(* Logix 5000 AddOnInstructionDefinition export AMCI_5034_PTO_AM_Preset_Encoder; software revision 37.00 *)

TYPE AMCI_5034_PTO_AM_Input_Data :
STRUCT
   ConnectionFaulted : DINT;
   MovingCW : BOOL;
   MovingCCW : BOOL;
   InHoldState : BOOL;
   Stopped : BOOL;
   AtHome : BOOL;
   Accelerating : BOOL;
   Decelerating : BOOL;
   MoveComplete : BOOL;
   HomeInvalid : BOOL;
   InvalidProfile : BOOL;
   PositionInvalid : BOOL;
   InputError : BOOL;
   CommandError : BOOL;
   ConfigurationError : BOOL;
   ModuleOK : BOOL;
   GeneralPurposeOutputStatus : BOOL;
   Input1Active : BOOL;
   Input2Active : BOOL;
   Input3Active : BOOL;
   Input4Active : BOOL;
   bit_20_reserved : BOOL;
   bit_21_reserved : BOOL;
   bit_22_reserved : BOOL;
   EncoderFollowerMode : BOOL;
   BlendMoveRunning : BOOL;
   BlendMoveAcknowledge : BOOL;
   MinimumRegistrationProgrammed : BOOL;
   EncoderMotionDirection : BOOL;
   MultipleInputsWithSameFunction : BOOL;
   FSCExceedsNumberOfDataBits : BOOL;
   AbsoluteEncoderSetupError : BOOL;
   bit_31_reserved : BOOL;
   CurrentPosition : DINT;
   EncoderPosition : DINT;
   CapturedPosition : DINT;
END_STRUCT
END_TYPE

TYPE AMCI_5034_PTO_AM_Output_Data :
STRUCT
   Command_Word : DINT;
   TargetPosition : DINT;
   TargetVelocity : UDINT;
   Acceleration : DINT;
   Deceleration : DINT;
END_STRUCT
END_TYPE

ADD_ON_INSTRUCTION AMCI_5034_PTO_AM_Preset_Encoder   (* revision 1.0, vendor AMCI, ExecuteEnableInFalse *)
// Revision note:
// 10/01/2025 initial release
// Help:
// PRESET_ENCODER: Preset Encoder Position to the Target Position value.
// AXIS INPUT DATA:  Input data from the AMCI 5034-PTO-AM.   Uses the AMCI_5034_PTO_Input_Data User Defined Data Type.
// AXIS OUTPUT DATA; Output data from the AOI to the AMCI 5034-PTO-AM.    Uses the AMCI_5034_PTO_Output_Data User Defined Data Type.
// TARGETPOSITION: Position to which the Encoder Position is to be set.
// EN (Enable) Set when rung is true, Reset when rung is false
// DN (Done) Set when command is sent to the motion device.  Reset when the rung is false.
// ER (Error) Set when a command or input error failed to clear.  Reset when the rung is false.
VAR_IN_OUT
   Axis_Input_Data : AMCI_5034_PTO_AM_Input_Data; {required}
   Axis_Output_Data : AMCI_5034_PTO_AM_Output_Data; {required}
END_VAR
VAR_INPUT
   TargetPosition : DINT; {required}
END_VAR
VAR_OUTPUT
   EN : BOOL; {visible}   // set when rung with AOI is true
   DN : BOOL; {access Read Only, visible}   // set when preset motor position command sent to motion axis
   ER : BOOL; {access Read Only, visible}   // set when input, command, or configuraiton error
END_VAR
VAR
   command_data_block : DINT[5];
        [0]   // Command Bits MSW
        [1]   // Target Position
        [2]   // Upper Target Position
        [3]   // Lower Target Position
        [4]   // Upper Programmed Speed
END_VAR

ROUTINE EnableInFalse   (* ladder *)
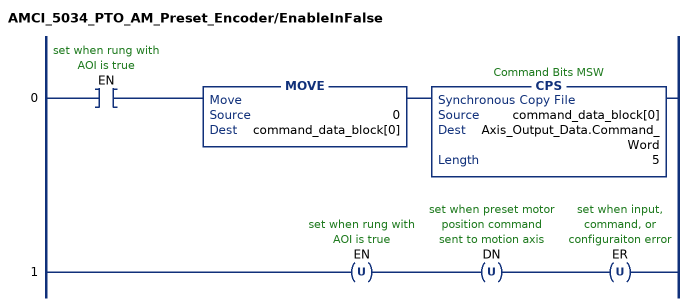
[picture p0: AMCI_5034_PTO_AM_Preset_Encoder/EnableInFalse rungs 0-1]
   0: XIC(EN)MOVE(0,command_data_block[0])CPS(command_data_block[0],Axis_Output_Data.Command_Word,5);
   1: OTU(EN)OTU(DN)OTU(ER);
END_ROUTINE

ROUTINE Logic   (* ladder *)
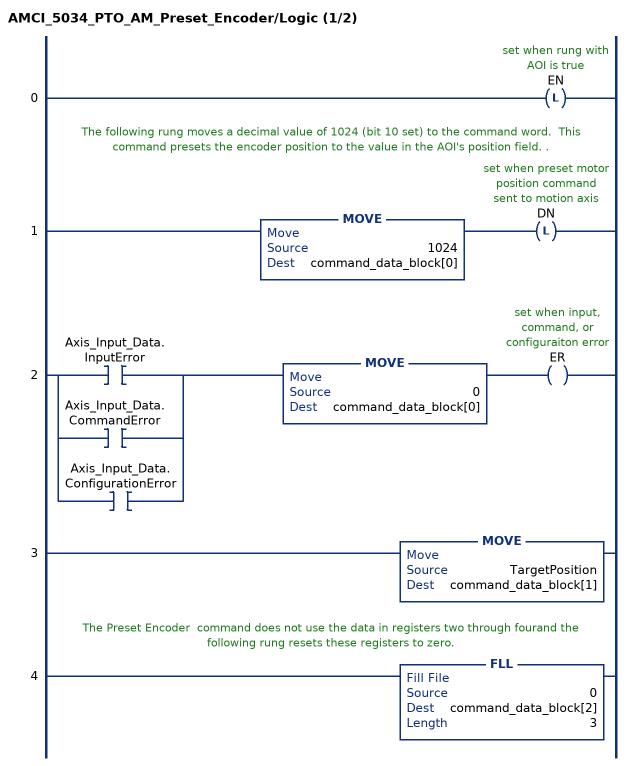
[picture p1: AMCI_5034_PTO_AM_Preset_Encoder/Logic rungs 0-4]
   0: OTL(EN);
   // The following rung moves a decimal value of 1024 (bit 10 set) to the command word.  This command presets the encoder position to the value in the AOI's position field. .
   1: MOVE(1024,command_data_block[0])OTL(DN);
   2: [XIC(Axis_Input_Data.InputError) ,XIC(Axis_Input_Data.CommandError) ,XIC(Axis_Input_Data.ConfigurationError) ]MOVE(0,command_data_block[0])OTE(ER);
   3: MOVE(TargetPosition,command_data_block[1]);
   // The Preset Encoder  command does not use the data in registers two through fourand the following rung resets these registers to zero.
   4: FLL(0,command_data_block[2],3);
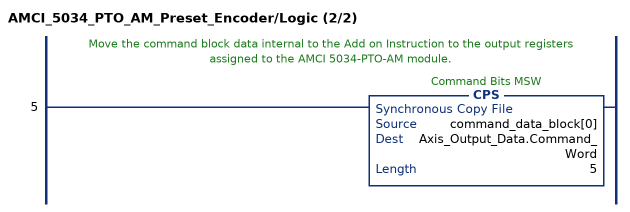
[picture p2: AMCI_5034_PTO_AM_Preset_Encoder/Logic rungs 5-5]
   // Move the command block data internal to the Add on Instruction to the output registers assigned to the AMCI 5034-PTO-AM module.
   5: CPS(command_data_block[0],Axis_Output_Data.Command_Word,5);
END_ROUTINE
END_ADD_ON_INSTRUCTION
